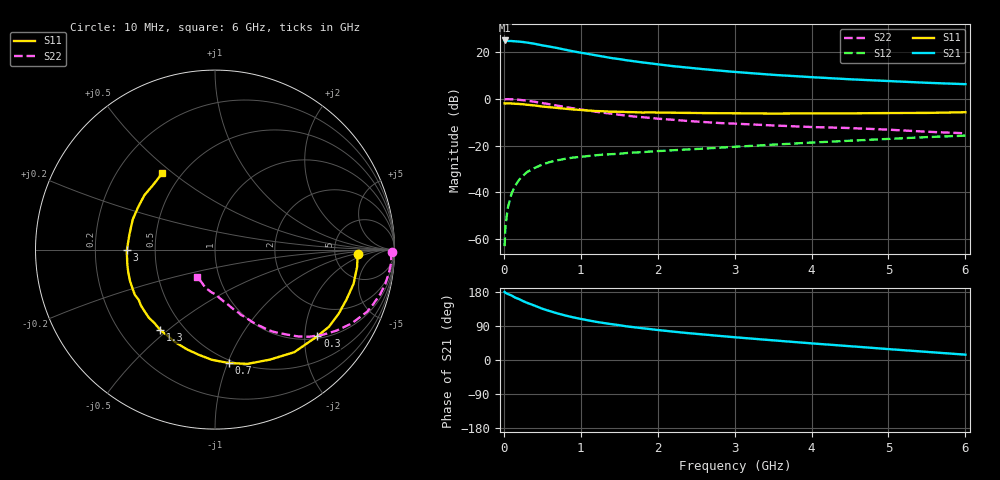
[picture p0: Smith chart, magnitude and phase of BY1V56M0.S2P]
! SIEMENS Small Signal Semiconductors
! BFY420
! Si NPN RF SIEGET Grounded Emitter Transistor in MICRO-X
! VCE = 1.5 V  IC = 6 mA
! Common Emitter S-Parameters:  October  1996
# GHz  S  MA  R  50
!  f  S11  S21  S12  S22
! GHz  MAG  ANG  MAG  ANG  MAG  ANG  MAG  ANG
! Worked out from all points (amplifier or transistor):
!   36 points, 10 MHz to 6 GHz, reference 50 ohm
!   highest |S21| = 25.0 dB at 10 MHz (marker M1)
!   |S21| within 3 dB of that: start of sweep to 655.2 MHz
!   unconditionally stable (mu >= 1): 2.939 GHz to end of sweep
!   at 250 MHz: K = 0.13, MSG = 28.6 dB, |S12| = -32.9 dB
!   at 1.4 GHz: K = 0.60, MSG = 20.6 dB, |S12| = -23.7 dB
!   at 6 GHz: K = 1.14, MAG = 8.8 dB, |S12| = -15.7 dB
!   S11 on the Smith chart (normalised r, x): 10 MHz: 8.80, -1.15; 300 MHz: 1.06, -2.31; 700 MHz: 0.48, -1.01; 1.3 GHz: 0.37, -0.47; 3 GHz: 0.34, -0.00; 6 GHz: 0.40, +0.46
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0.01  0.799 -1.7  17.8 179.7  0.0007 96.4  0.9872 -0.7
0.02  0.7952 -3.1  17.71 177.5  0.0018 84.7  0.9805 -1.4
0.05  0.7975 -7.0  17.37 174.4  0.0045 89.1  0.9849 -3.9
0.1  0.7951 -13.9  17.31 170.3  0.0094 84.1  0.9775 -7.7
0.15  0.7836 -20.7  17.03 164.4  0.014 78.0  0.9676 -11.5
0.2  0.7763 -27.3  16.79 160.5  0.0186 76.5  0.9535 -15.1
0.25  0.767 -34.0  16.49 155.4  0.0227 72.1  0.9336 -18.8
0.3  0.7473 -40.2  16.05 151.0  0.0269 69.6  0.9165 -22.1
0.4  0.7224 -52.3  15.11 143.5  0.0331 64.0  0.8652 -28.4
0.5  0.685 -63.5  13.98 135.3  0.0392 59.7  0.8138 -33.7
0.6  0.6619 -74.1  13.1 128.9  0.0445 55.3  0.7624 -38.6
0.7  0.6371 -82.9  12.21 122.8  0.0483 52.2  0.7143 -42.8
0.9  0.5928 -98.8  10.43 112.6  0.0552 47.0  0.6273 -49.2
1.1  0.5622 -112.9  9.136 104.5  0.0597 43.9  0.5593 -54.8
1.3  0.5418 -124.5  7.993 97.6  0.0642 41.3  0.5024 -58.8
1.6  0.5213 -139.1  6.683 88.7  0.0692 39.4  0.4366 -64.0
2.2  0.5049 -159.6  5.017 74.9  0.0793 37.2  0.3563 -71.9
3  0.4913 -179.5  3.775 60.1  0.0941 35.4  0.2948 -80.1
3.5  0.4841 169.8  3.271 51.9  0.1044 33.9  0.2694 -84.9
4.5  0.4889 151.2  2.625 36.4  0.1269 29.1  0.2368 -95.6
5.5  0.4998 132.8  2.207 21.4  0.1515 22.7  0.1975 -112.1
6  0.5171 124.6  2.063 14.1  0.1632 19.0  0.183 -122.9
